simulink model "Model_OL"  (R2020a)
settings: Solver=FixedStepAuto  StartTime=0.0  StopTime=tsim  FixedStep=0.1  RelTol=1e-5
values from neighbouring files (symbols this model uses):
  C = Fc*cpc/(Fh*cph)    [calcblock.m]    (also in calcblock2.m; calcblock3.m; eNTU.m = m.c*cp.c/(m.h*cp.h); Main.m = [zeros(1,2*N-1),1])
  d_tstep = 300    [Main.m]    (also in Main_OL.m = 3000; runTestCalcBlk.m; runTransf.m = [500; 50000; 70000; 130000; 50000; 50000]; runTransfOL.m = [500 5000 7000 13000])
  dFc = 0    [Main.m]    (also in Main_OL.m = dist(i); runTransfOL.m = -0.5)
  dFh = 0;0.2*Fh    [Main.m]    (also in runTransf.m = 2; runTransfOL.m = 0)
  dTcin = 2    [Main.m]    (also in runTransf.m = 0; runTransfOL.m = 0)
  dThin = 0;2    [Main.m]    (also in runTransf.m = 0; runTransfOL.m = 0)
  Fc0 = 5    [Main.m]    (also in Main_OL.m; runTestCalcBlk.m; runTransf.m; runTransfOL.m)
  Fh = d(1)    [calcblock.m]    (also in calcblock2.m; calcblock3.m; HEXode.m; Main.m = 3)
  nd = size(d0,2)    [Main.m]    (also in Main_OL.m; runTestCalcBlk.m; runTransf.m = size(d0,1); runTransfOL.m)
  np = size(p,2)    [Main.m]    (also in Main_OL.m; runTestCalcBlk.m; runH2Psim.m = length(param); runTransf.m)
  nu = 1    [Main.m]    (also in Main_OL.m; runTestCalcBlk.m; runH2Psim.m = length(u0); runTransf.m)
  nx = size(x0,1)    [Main.m]    (also in Main_OL.m; runTestCalcBlk.m; H2P_Turbine_driven.m = param(end); runTD.m = length(x0))
  p = [N, Fc0, rhoc, rhoh,U,A,cpc,cph]    [Main.m]    (also in Main_OL.m; runTestCalcBlk.m; NonlinearMap.m = [U;A;Fc(i);Fh;cpc;cph;Tcin;Thin]; runTransf.m = [N, Fc0, rhoc, rhoh, U0, A,cpc,cph])
  tau = 10    [Main.m]    (also in Main_OL.m = 130; runTransf.m = [100;310;400]; runTransfOL.m = [100;310;400])
  Tcin = d(2)    [calcblock.m]    (also in calcblock2.m; calcblock3.m; HEXode.m; Main.m = 293.15)
  theta = 0    [Main.m]    (also in Main_OL.m = 40; runTransf.m = [40;60;60]; runTransfOL.m = [40;60;60]; BaseCase.m)
  Thin = d(3)    [calcblock.m]    (also in calcblock2.m; calcblock3.m; HEXode.m; Main.m = 343.15)
  tstep = 100    [Main.m]    (also in Main_OL.m = 500; runTransf.m = 10000; runTransfOL.m)
  x0 = [Tcend(1:N)'; Thend(1:N)']    [Main.m]    (also in Main_OL.m; runTestCalcBlk.m; runTD.m = [TE0;TD0;TSh0;MD0; MSh0;w0;TA0;0;0;0;0;0;0;0;0;0]; runBD.m = [TE0;TD0;TSh0;MD0; MSh0;w0;TA0;0;0;0;0;0;0;0;0;0])
undefined symbols (not defined in the file or in its folder): HEXode

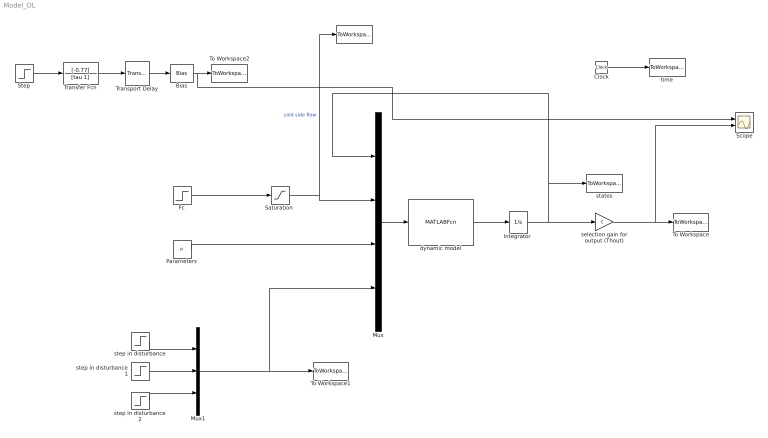
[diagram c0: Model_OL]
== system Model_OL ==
  " " : ToWorkspace  VariableName=uc  SampleTime=-1
  Bias : Bias  Bias=x0(end)
  Clock : Clock
  Fc : Step  Time=tstep  Before=Fc0  After=Fc0+dFc  SampleTime=0
  "Integrator " : Integrator  InitialCondition=x0
  Mux : Mux
  Mux1 : Mux  Inputs=3
  Parameters : Constant  Value=p
  "Saturation " : Saturate  UpperLimit=inf  LowerLimit=0
  Scope : Scope  NumInputPorts=2
  Step : Step  Time=tstep  After=dFc  SampleTime=0
  To Workspace : ToWorkspace  VariableName=Thout  SampleTime=-1
  To Workspace1 : ToWorkspace  VariableName=dsim  SampleTime=-1
  To Workspace2 : ToWorkspace  VariableName=ytf  SampleTime=-1
  Transfer Fcn : TransferFcn  Numerator=[-0.77]  Denominator=[tau 1]
  Transport Delay : TransportDelay  DelayTime=theta
  dynamic model : MATLABFcn  MATLABFcn=HEXode(u(1:nx),u(nx+1:nx+nu),u(nx+nu+1:nx+nu+np),u(nx+nu+np+1:nx+nu+np+nd))  OutputDimensions=nx  Output1D=off
  selection gain for output (Thout) : Gain  Gain=C  Multiplication=Matrix(K*u)
  states : ToWorkspace  VariableName=T  SampleTime=-1
  step in disturbance : Step  Time=d_tstep(1)  Before=Fh  After=Fh+dFh  SampleTime=0
  step in disturbance1 : Step  Time=d_tstep(2)  Before=Tcin  After=Tcin+dTcin  SampleTime=0
  step in disturbance2 : Step  Time=d_tstep(3)  Before=Thin  After=Thin+dThin  SampleTime=0
  time : ToWorkspace  VariableName=t  SampleTime=-1
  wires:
  dynamic model/1 -> "Integrator "/1
  "Integrator "/1 -> states/1, Mux/1, selection gain for output (Thout)/1
  Mux/1 -> dynamic model/1
  Clock/1 -> time/1
  Parameters/1 -> Mux/3
  "Saturation "/1 -> Mux/2, " "/1  "cold side flow"
  selection gain for output (Thout)/1 -> Scope/2, To Workspace/1
  Transfer Fcn/1 -> Transport Delay/1
  Transport Delay/1 -> Bias/1
  Fc/1 -> "Saturation "/1
  Step/1 -> Transfer Fcn/1
  Bias/1 -> Scope/1, To Workspace2/1
  Mux1/1 -> Mux/4, To Workspace1/1
  step in disturbance2/1 -> Mux1/3
  step in disturbance1/1 -> Mux1/2
  step in disturbance/1 -> Mux1/1
